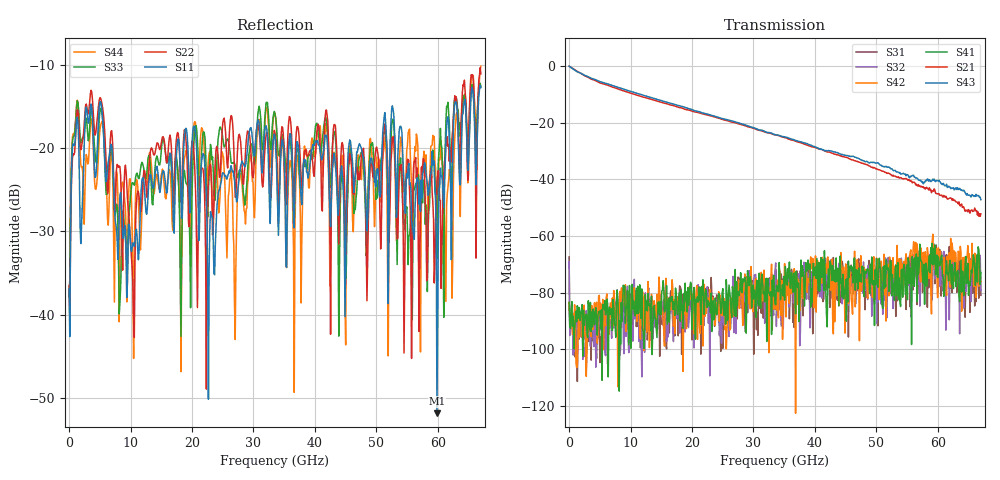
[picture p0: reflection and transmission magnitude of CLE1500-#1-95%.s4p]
!Keysight Technologies,N5247B,US50470101,A.16.20.02
!Date: Thursday, March 13, 2025 10:34:36
!Correction: S11(C  4-Port  )
!S12(C  4-Port  )
!S13(C  4-Port  )
!S14(C  4-Port  )
!S21(C  4-Port  )
!S22(C  4-Port  )
!S23(C  4-Port  )
!S24(C  4-Port  )
!S31(C  4-Port  )
!S32(C  4-Port  )
!S33(C  4-Port  )
!S34(C  4-Port  )
!S41(C  4-Port  )
!S42(C  4-Port  )
!S43(C  4-Port  )
!S44(C  4-Port  )
!S4P File: Measurements: <S11,S12,S13,S14>,
!<S21,S22,S23,S24>,
!<S31,S32,S33,S34>,
!<S41,S42,S43,S44>:
# Hz S  dB  R 50
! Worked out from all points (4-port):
!   601 points, 10 MHz to 67 GHz, reference 50 ohm
!   strongest paths, dB at 10 MHz, 16.76 GHz, 33.51 GHz, 50.25 GHz, 67 GHz:
!     S43: 0.0, -13.2, -24.2, -34.1, -47.2
!     S21: 0.0, -13.8, -24.3, -36.5, -52.2
!     S41: -83.4, -81.4, -83.9, -78.1, -72.9
!     S42: -83.6, -75.4, -85.8, -71.5, -76.1
!     S32: -69.1, -87.2, -72.4, -83.4, -79.3
!     S31: -67.3, -78.2, -85.9, -91.7, -80.9
!   lowest |S11| = -51.8 dB at 59.85 GHz (marker M1), VSWR 1.01, Z = 50.2 + j0.17 ohm
!   |S11| at or under -10 dB: start of sweep to end of sweep
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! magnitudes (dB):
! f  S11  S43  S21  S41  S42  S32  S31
! 10 MHz  -36.9  0.0  0.0  -83.4  -83.6  -69.1  -67.3
! 3.583 GHz  -14.7  -4.3  -4.6  -93.7  -95.5  -95.7  -103.8
! 10.39 GHz  -31.4  -9.1  -9.8  -85.7  -80.2  -97.1  -84.1
! 15.19 GHz  -22.9  -12.3  -12.9  -79.1  -87.0  -87.3  -90.9
! 52.6 GHz  -14.9  -36.4  -38.8  -73.5  -72.8  -73.9  -76.4
! 59.85 GHz  -51.8  -40.4  -45.0  -66.7  -70.8  -67.2  -70.3
! 67 GHz  -12.7  -47.2  -52.2  -72.9  -76.1  -79.3  -80.9
